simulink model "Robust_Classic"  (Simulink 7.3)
settings: Solver=ode45  StartTime=0.0  StopTime=80  RelTol=1e-3
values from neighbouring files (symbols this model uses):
  d2r = 1/r2d    (= 0.0174532925199)    [init.m]    (also in freq.m; frequ.m; init_lat.m; pl.m)
  r2d = 180/pi    (= 57.2957795131)    [init.m]    (also in freq.m; frequ.m; init_lat.m; pl.m)
undefined symbols (not defined in the file or in its folder): Avu, Bvu, Cvu, Dvu

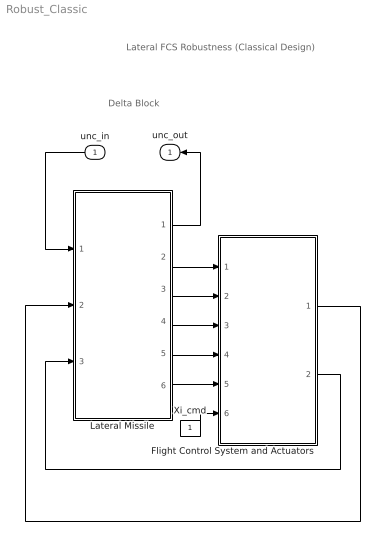
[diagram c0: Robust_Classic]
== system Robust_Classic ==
  note: Lateral FCS Robustness (Classical Design)
  note: Delta Block
  unc_in : Inport  OutDataType=sfix(16)  OutScaling=2^0
  Flight Control System and Actuators : Subsystem
  Lateral Missile : Subsystem
  Xi_cmd : Constant  OutDataType=fixdt(1, 16)  OutScaling=2^0
  unc_out : Outport
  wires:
  Lateral Missile/2(p) -> Flight Control System and Actuators/1(p)
  Lateral Missile/3(phi) -> Flight Control System and Actuators/2(phi)
  Lateral Missile/4(r) -> Flight Control System and Actuators/3(r)
  Lateral Missile/5(psi) -> Flight Control System and Actuators/4(psi)
  Lateral Missile/6(Ny) -> Flight Control System and Actuators/5(Nym)
  Flight Control System and Actuators/2(d-ruddr) -> Lateral Missile/3(drud)
  Flight Control System and Actuators/1(d-ailer) -> Lateral Missile/2(dail)
  Lateral Missile/1(unc_out) -> unc_out/1
  unc_in/1 -> Lateral Missile/1(unc-in)
  Xi_cmd/1 -> Flight Control System and Actuators/6(Xi_Cmd)

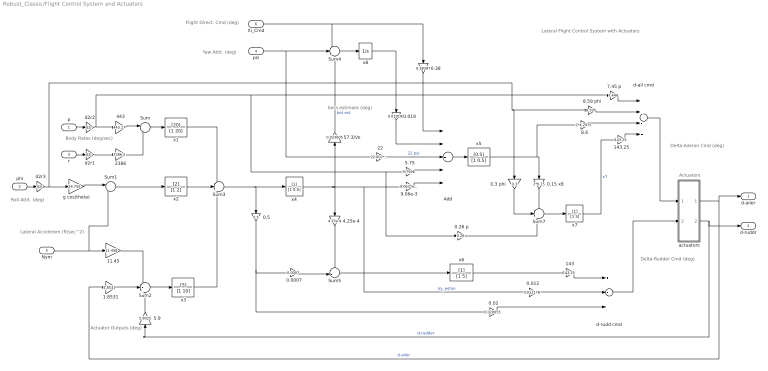
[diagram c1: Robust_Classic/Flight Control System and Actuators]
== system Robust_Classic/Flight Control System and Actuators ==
  note: Body Rates (deg/sec)
  note: Delta-Rudder Cmd (deg)
  note: Delta-Aileron Cmd (deg)
  note: Lateral Accelerom (ft/sec^2)
  note: Actuator Outputs (deg)
  note: Roll Attit. (deg)
  note: Yaw Attit. (deg)
  note: Flight Direct. Cmd (deg)
  note: beta estimate (deg)
  note: Actuators
  note: Lateral Flight Control System with Actuators
  p : Inport  OutDataType=fixdt(1, 16)  OutScaling=2^0
  phi : Inport  Port=2  OutDataType=fixdt(1, 16)  OutScaling=2^0
  r : Inport  Port=3  OutDataType=fixdt(1, 16)  OutScaling=2^0
  psi : Inport  Port=4  OutDataType=fixdt(1, 16)  OutScaling=2^0
  Nym : Inport  Port=5  OutDataType=fixdt(1, 16)  OutScaling=2^0
  Xi_Cmd : Inport  Port=6  OutDataType=fixdt(1, 16)  OutScaling=2^0
  0.0007 : Gain  Gain=0.0007  ParameterDataType=fixdt(1, 16)  ParameterScaling=2^0  OutDataType=fixdt(1, 16)  OutScaling=2^0
  0.012 : Gain  Gain=0.012176  ParameterDataType=fixdt(1, 16)  ParameterScaling=2^0  OutDataType=fixdt(1, 16)  OutScaling=2^0
  0.019 : Gain  Gain=0.019199  ParameterDataType=fixdt(1, 16)  ParameterScaling=2^0  OutDataType=fixdt(1, 16)  OutScaling=2^0
  0.02 : Gain  Gain=0.020055  ParameterDataType=fixdt(1, 16)  ParameterScaling=2^0  OutDataType=fixdt(1, 16)  OutScaling=2^0
  0.15 x8 : Gain  Gain=2*0.15  ParameterDataType=fixdt(1, 16)  ParameterScaling=2^0  OutDataType=fixdt(1, 16)  OutScaling=2^0
  0.26 p : Gain  Gain=0.26  ParameterDataType=fixdt(1, 16)  ParameterScaling=2^0  OutDataType=fixdt(1, 16)  OutScaling=2^0
  0.3 phi : Gain  Gain=0.3  ParameterDataType=fixdt(1, 16)  ParameterScaling=2^0  OutDataType=fixdt(1, 16)  OutScaling=2^0
  0.38 : Gain  Gain=0.38397  ParameterDataType=fixdt(1, 16)  ParameterScaling=2^0  OutDataType=fixdt(1, 16)  OutScaling=2^0
  0.5 : Gain  Gain=0.5  ParameterDataType=fixdt(1, 16)  ParameterScaling=2^0  OutDataType=fixdt(1, 16)  OutScaling=2^0
  1.8531 : Gain  Gain=1.8531  ParameterDataType=fixdt(1, 16)  ParameterScaling=2^0  OutDataType=fixdt(1, 16)  OutScaling=2^0
  11.45 : Gain  Gain=11.458  ParameterDataType=fixdt(1, 16)  ParameterScaling=2^0  OutDataType=fixdt(1, 16)  OutScaling=2^0
  143 : Gain  Gain=143.25  ParameterDataType=fixdt(1, 16)  ParameterScaling=2^0  OutDataType=fixdt(1, 16)  OutScaling=2^0
  143.25 : Gain  Gain=143.25  ParameterDataType=fixdt(1, 16)  ParameterScaling=2^0  OutDataType=fixdt(1, 16)  OutScaling=2^0
  22 : Gain  Gain=22.002*d2r  ParameterDataType=fixdt(1, 16)  ParameterScaling=2^0  OutDataType=fixdt(1, 16)  OutScaling=2^0
  2386 : Gain  Gain=2386.5  ParameterDataType=fixdt(1, 16)  ParameterScaling=2^0  OutDataType=fixdt(1, 16)  OutScaling=2^0
  4.25e-4 : Gain  Gain=4.25e-4  ParameterDataType=fixdt(1, 16)  ParameterScaling=2^0  OutDataType=fixdt(1, 16)  OutScaling=2^0
  443 : Gain  Gain=443.17  ParameterDataType=fixdt(1, 16)  ParameterScaling=2^0  OutDataType=fixdt(1, 16)  OutScaling=2^0
  5.75 : Gain  Gain=5.7596  ParameterDataType=fixdt(1, 16)  ParameterScaling=2^0  OutDataType=fixdt(1, 16)  OutScaling=2^0
  5.9 : Gain  Gain=5.9025  ParameterDataType=fixdt(1, 16)  ParameterScaling=2^0  OutDataType=fixdt(1, 16)  OutScaling=2^0
  57.3/Vo : Gain  Gain=0.023605  ParameterDataType=fixdt(1, 16)  ParameterScaling=2^0  OutDataType=fixdt(1, 16)  OutScaling=2^0
  7.45 p : Gain  Gain=7.449  ParameterDataType=fixdt(1, 16)  ParameterScaling=2^0  OutDataType=fixdt(1, 16)  OutScaling=2^0
  8.59 phi : Gain  Gain=8.595  ParameterDataType=fixdt(1, 16)  ParameterScaling=2^0  OutDataType=fixdt(1, 16)  OutScaling=2^0
  8.6 : Gain  Gain=2*4.2975  ParameterDataType=fixdt(1, 16)  ParameterScaling=2^0  OutDataType=fixdt(1, 16)  OutScaling=2^0
  "9.06e-3 " : Gain  Gain=9.0637e-3  ParameterDataType=fixdt(1, 16)  ParameterScaling=2^0  OutDataType=fixdt(1, 16)  OutScaling=2^0
  Add : Sum  Inputs=++---  OutDataType=fixdt(1, 16)  OutScaling=2^-10
  Sum : Sum  Inputs=|-+  OutDataType=fixdt(1, 16)  OutScaling=2^0
  Sum1 : Sum  Inputs=|++  OutDataType=fixdt(1, 16)  OutScaling=2^0
  Sum2 : Sum  Inputs=-++  OutDataType=fixdt(1, 16)  OutScaling=2^0
  Sum3 : Sum  Inputs=-++  OutDataType=fixdt(1, 16)  OutScaling=2^0
  Sum4 : Sum  Inputs=+--  OutDataType=fixdt(1, 16)  OutScaling=2^0
  Sum5 : Sum  Inputs=--|  OutDataType=fixdt(1, 16)  OutScaling=2^0
  Sum7 : Sum  Inputs=-++  OutDataType=fixdt(1, 16)  OutScaling=2^0
  actuators : Subsystem
  d-ail cmd : Sum  Inputs=++-+  OutDataType=fixdt(1, 16)  OutScaling=2^-10
  d-rudd cmd : Sum  Inputs=+--  OutDataType=fixdt(1, 16)  OutScaling=2^-10
  d2r1 : Gain  Gain=d2r  ParameterDataType=fixdt(1, 16)  ParameterScaling=2^0  OutDataType=fixdt(1, 16)  OutScaling=2^0
  d2r2 : Gain  Gain=d2r  ParameterDataType=fixdt(1, 16)  ParameterScaling=2^0  OutDataType=fixdt(1, 16)  OutScaling=2^0
  d2r3 : Gain  Gain=d2r  ParameterDataType=fixdt(1, 16)  ParameterScaling=2^0  OutDataType=fixdt(1, 16)  OutScaling=2^0
  g cos(theta) : Gain  Gain=24.755  ParameterDataType=fixdt(1, 16)  ParameterScaling=2^0  OutDataType=fixdt(1, 16)  OutScaling=2^0
  x1 : TransferFcn  Numerator=[20]  Denominator=[1 20]
  x2 : TransferFcn  Numerator=[2]  Denominator=[1 2]
  x3 : TransferFcn  Numerator=[5]  Denominator=[1 10]
  x4 : TransferFcn  Denominator=[1 0.5]
  x5 : TransferFcn  Numerator=[0.5]  Denominator=[1 0.5]
  x6 : TransferFcn  Denominator=[1 5]
  x7 : TransferFcn  Denominator=[1 5]
  x8 : Integrator
  d-ailer : Outport  OutDataType=fixdt(1, 16)  OutScaling=2^0
  d-ruddr : Outport  Port=2  OutDataType=fixdt(1, 16)  OutScaling=2^0
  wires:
  0.5/1 -> 0.02/1, 0.0007/1
  d-rudd cmd/1 -> actuators/2(dr)
  0.02/1 -> d-rudd cmd/3
  0.012/1 -> d-rudd cmd/2
  x6/1 -> 143/1
  143/1 -> d-rudd cmd/1
  d-ail cmd/1 -> actuators/1(da)
  7.45 p/1 -> d-ail cmd/1
  8.59 phi/1 -> d-ail cmd/2
  143.25/1 -> d-ail cmd/4
  x7/1 -> 143.25/1  "x7"
  8.6/1 -> d-ail cmd/3
  0.3 phi/1 -> Sum7/2
  0.26 p/1 -> Sum7/3
  0.15 x8/1 -> Sum7/1
  Sum7/1 -> x7/1
  x5/1 -> 8.6/1, 0.15 x8/1
  5.75/1 -> Add/4
  22/1 -> Add/3  "22 psi"
  0.019/1 -> Add/2
  x8/1 -> 0.019/1
  Add/1 -> x5/1
  "9.06e-3 "/1 -> Add/5
  0.38/1 -> Add/1
  Sum5/1 -> x6/1
  0.0007/1 -> Sum5/2
  4.25e-4/1 -> Sum5/1
  Nym/1 -> Sum1/2, 11.45/1
  Sum4/1 -> x8/1
  57.3/Vo/1 -> Sum4/3  "bet est"
  x4/1 -> 0.012/1, "9.06e-3 "/1, 4.25e-4/1, 57.3/Vo/1  "Vy_estim"
  psi/1 -> Sum4/2, 22/1
  Xi_Cmd/1 -> 0.38/1, Sum4/1
  Sum3/1 -> 0.5/1, x4/1
  x3/1 -> Sum3/3
  x2/1 -> Sum3/2
  x1/1 -> Sum3/1
  Sum2/1 -> x3/1
  5.9/1 -> Sum2/3
  1.8531/1 -> Sum2/2
  11.45/1 -> Sum2/1
  phi/1 -> d2r3/1
  g cos(theta)/1 -> Sum1/1
  Sum1/1 -> x2/1
  2386/1 -> Sum/2
  r/1 -> d2r1/1
  p/1 -> d2r2/1
  443/1 -> Sum/1
  Sum/1 -> x1/1
  actuators/1("da ") -> d-ailer/1, 1.8531/1  "d-ailer"
  actuators/2("dr ") -> d-ruddr/1, 5.9/1  "d-rudder"
  d2r3/1 -> 8.59 phi/1, 0.3 phi/1, g cos(theta)/1
  d2r2/1 -> 7.45 p/1, 0.26 p/1, 5.75/1, 443/1
  d2r1/1 -> 2386/1

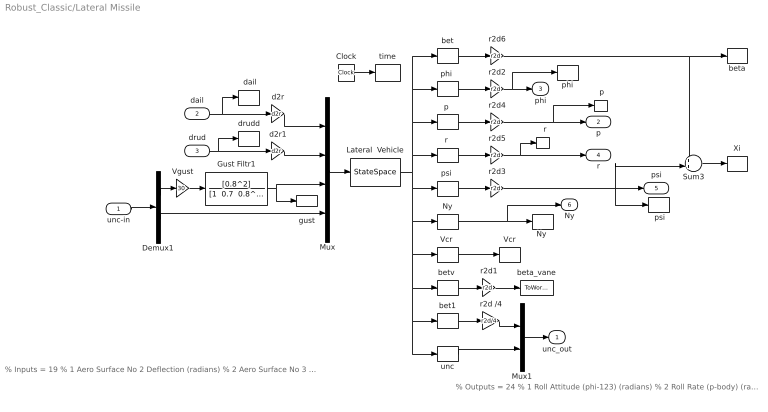
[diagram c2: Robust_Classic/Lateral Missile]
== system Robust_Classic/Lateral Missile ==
  note: % Outputs = 24 % 1 Roll Attitude (phi-123) (radians) % 2 Roll Rate (p-body) (rad/sec) % 3 Yaw Attitude (psi-123) (radians) % 4 Yaw Rate (r-body) (rad/sec) % 5 Angle of sideslip, beta, (radian) % 6 Cross Range Velocity (Vcr) (ft/sec) % 7 Accelerom # 1, (along Y), (ft/sec^2) % 8 Beta Sensed at Vane # 1 (radian) % 9 Cl_beta : -17.647 % Variation % 10 Cn_beta : 17.565 % Variation % 11 Cy_beta : -26.087 % Variation % 12 Cn_p : 36.023 % Variation % 13 Cn_r : -19.802 % Variation % 14 Cl_p : -20.576 % Variation % 15 Cl_r : 37.622 % Variation % 16 I_xx : 7.384 % Variation % 17 I_zz : 2.411 % Variation % 18 Xcg locat: 1.909 % Variation % 19 Cy_surf 2: 45.455 % Variation % 20 Cl_surf 2: -15.289 % Variation % 21 Cn_surf 2: -28.571 % Variation % 22 Cy_surf 3: 29.412 % Variation % 23 Cl_surf 3: 16.819 % Variation % 24 Cn_surf 3: -28.571 % Variation
  note: % Inputs = 19 % 1 Aero Surface No 2 Deflection (radians) % 2 Aero Surface No 3 Deflection (radians) % 3 Wind Gust Azim, Elev Angles=( 45.0 90.0) (deg) % 4 Cl_beta : -17.647 % Variation % 5 Cn_beta : 17.565 % Variation % 6 Cy_beta : -26.087 % Variation % 7 Cn_p : 36.023 % Variation % 8 Cn_r : -19.802 % Variation % 9 Cl_p : -20.576 % Variation % 10 Cl_r : 37.622 % Variation % 11 I_xx : 7.384 % Variation % 12 I_zz : 2.411 % Variation % 13 Xcg locat: 1.909 % Variation % 14 Cy_surf 2: 45.455 % Variation % 15 Cl_surf 2: -15.289 % Variation % 16 Cn_surf 2: -28.571 % Variation % 17 Cy_surf 3: 29.412 % Variation % 18 Cl_surf 3: 16.819 % Variation % 19 Cn_surf 3: -28.571 % Variation
  unc-in : Inport
  dail : Inport  Port=2
  drud : Inport  Port=3
  "  r" : ToWorkspace  VariableName=r  SampleTime=-1  SaveFormat=Array
  " Ny " : Selector  InputPortWidth=24  IndexOptions=Index vector (dialog)  Indices=[7]  OutputSizes=1
  " Xi " : ToWorkspace  VariableName=Xi  SampleTime=-1  SaveFormat=Array
  " dail" : ToWorkspace  VariableName=dail  SampleTime=-1  SaveFormat=Array
  " drudd " : ToWorkspace  VariableName=drud  SampleTime=-1  SaveFormat=Array
  " p" : ToWorkspace  VariableName=p  SampleTime=-1  SaveFormat=Array
  " phi " : ToWorkspace  VariableName=phi  SampleTime=-1  SaveFormat=Array
  " psi" : ToWorkspace  VariableName=psi  SampleTime=-1  SaveFormat=Array
  Clock : Clock
  Demux1 : Demux  Outputs=[1, 16]
  Gust Filtr1 : TransferFcn  Numerator=[0.8^2]  Denominator="[1  0.7  0.8^2]"
  Lateral  Vehicle : StateSpace  A=Avu  B=Bvu  C=Cvu  D=Dvu
  Mux : Mux  Inputs=[1, 1, 1, 16]
  Mux1 : Mux  Inputs="[1,  16]"
  "Ny " : ToWorkspace  VariableName=Ny  SampleTime=-1  SaveFormat=Array
  Sum3 : Sum  Inputs=++|  OutDataType=fixdt(1, 16)  OutScaling=2^0
  Vcr : ToWorkspace  VariableName=Vcr  SampleTime=-1  SaveFormat=Array
  "Vcr " : Selector  InputPortWidth=24  IndexOptions=Index vector (dialog)  Indices=[6]  OutputSizes=1
  Vgust : Gain  Gain=30  ParameterDataType=fixdt(1, 16)  ParameterScaling=2^0  OutDataType=fixdt(1, 16)  OutScaling=2^0
  bet : Selector  InputPortWidth=24  IndexOptions=Index vector (dialog)  Indices=[5]  OutputSizes=1
  bet1 : Selector  InputPortWidth=24  IndexOptions=Index vector (dialog)  Indices=[5]  OutputSizes=1
  beta : ToWorkspace  VariableName=beta  SampleTime=-1  SaveFormat=Array
  beta_vane : ToWorkspace  VariableName=beta_vn  SampleTime=-1  SaveFormat=Array
  "betv " : Selector  InputPortWidth=24  IndexOptions=Index vector (dialog)  Indices=[8]  OutputSizes=1
  d2r : Gain  Gain=d2r  ParameterDataType=fixdt(1, 16)  ParameterScaling=2^0  OutDataType=fixdt(1, 16)  OutScaling=2^0
  d2r1 : Gain  Gain=d2r  ParameterDataType=fixdt(1, 16)  ParameterScaling=2^0  OutDataType=fixdt(1, 16)  OutScaling=2^0
  gust : ToWorkspace  VariableName=Vgst  SampleTime=-1  SaveFormat=Array
  "p " : Selector  InputPortWidth=24  IndexOptions=Index vector (dialog)  Indices=[2]  OutputSizes=1
  "phi " : Selector  InputPortWidth=24  IndexOptions=Index vector (dialog)  Indices=[1]  OutputSizes=1
  "psi " : Selector  InputPortWidth=24  IndexOptions=Index vector (dialog)  Indices=[3]  OutputSizes=1
  "r " : Selector  InputPortWidth=24  IndexOptions=Index vector (dialog)  Indices=[4]  OutputSizes=1
  r2d /4 : Gain  Gain=r2d/4  ParameterDataType=fixdt(1, 16)  ParameterScaling=2^0  OutDataType=fixdt(1, 16)  OutScaling=2^0
  r2d{1..6} (6 alike) : Gain  Gain=r2d  ParameterDataType=fixdt(1, 16)  ParameterScaling=2^0  OutDataType=fixdt(1, 16)  OutScaling=2^0
  time : ToWorkspace  VariableName=time  SampleTime=-1  SaveFormat=Array
  unc : Selector  InputPortWidth=24  IndexOptions=Index vector (dialog)  Indices=[9:24]  OutputSizes=1
  unc_out : Outport
  p : Outport  Port=2
  phi : Outport  Port=3
  r : Outport  Port=4
  psi : Outport  Port=5
  Ny : Outport  Port=6
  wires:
  Mux/1 -> Lateral  Vehicle/1
  Lateral  Vehicle/1 -> "Vcr "/1, "betv "/1, unc/1, bet1/1, " Ny "/1, "psi "/1, bet/1, "phi "/1, "p "/1, "r "/1
  dail/1 -> d2r/1, " dail"/1
  drud/1 -> d2r1/1, " drudd "/1
  Sum3/1 -> " Xi "/1
  r2d2/1 -> phi/1, " phi "/1
  r2d3/1 -> psi/1, Sum3/2, " psi"/1
  r2d4/1 -> p/1, " p"/1
  r2d5/1 -> r/1, "  r"/1
  d2r1/1 -> Mux/2
  r2d1/1 -> beta_vane/1
  Clock/1 -> time/1
  r2d6/1 -> Sum3/1, beta/1
  bet/1 -> r2d6/1
  "phi "/1 -> r2d2/1
  "p "/1 -> r2d4/1
  "r "/1 -> r2d5/1
  "psi "/1 -> r2d3/1
  " Ny "/1 -> Ny/1, "Ny "/1
  "Vcr "/1 -> Vcr/1
  "betv "/1 -> r2d1/1
  d2r/1 -> Mux/1
  unc-in/1 -> Demux1/1
  Demux1/1 -> Vgust/1
  Demux1/2 -> Mux/4
  Vgust/1 -> Gust Filtr1/1
  bet1/1 -> r2d /4/1
  unc/1 -> Mux1/2
  Mux1/1 -> unc_out/1
  Gust Filtr1/1 -> Mux/3, gust/1
  r2d /4/1 -> Mux1/1

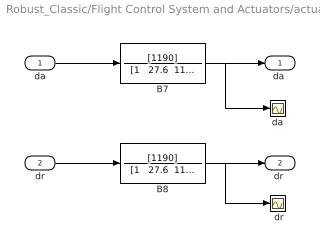
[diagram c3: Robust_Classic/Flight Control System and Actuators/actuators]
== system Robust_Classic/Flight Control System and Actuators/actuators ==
  da : Inport
  dr : Inport  Port=2
  " da " : Scope
  " dr" : Scope
  B7 : TransferFcn  Numerator=[1190]  Denominator="[1   27.6  1190]"
  B8 : TransferFcn  Numerator=[1190]  Denominator="[1   27.6  1190]"
  "da " : Outport
  "dr " : Outport  Port=2
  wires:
  B8/1 -> " dr"/1, "dr "/1
  dr/1 -> B8/1
  B7/1 -> " da "/1, "da "/1
  da/1 -> B7/1
